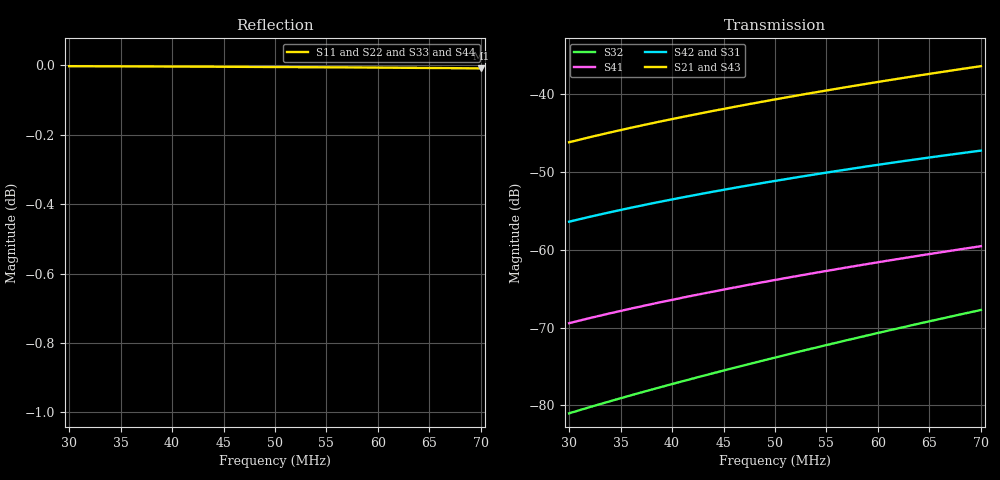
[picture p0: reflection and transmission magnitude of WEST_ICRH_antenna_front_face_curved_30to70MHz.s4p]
! Touchstone file exported from HFSS 2020.2.0
!  File:  C:/Users/JH218595/Documents/ICRH/WEST/HFSS_antenna_front_face/WEST_ICRH_front_face.aedt
!  Generated:  10:17:14  ao%xFBt 03, 2020
!  Design:  Front Face Curved
!  Project:  WEST_ICRH_front_face
!  Setup:  Setup1
!  Solution:  Sweep_operationnal
! Variables:
!  $epsr_dielectric = 1
!  $shift_X = 50mm
!  dphi = -180deg
!Data is not renormalized
# GHZ S MA
! Terminal data exported
! Port[1] = 1
! Port[2] = 2
! Port[3] = 3
! Port[4] = 4
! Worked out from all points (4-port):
!   4001 points, 30 MHz to 70 MHz, reference per port
!   strongest paths, dB at 30 MHz, 40 MHz, 50 MHz, 60 MHz, 70 MHz:
!     S21: -46.2, -43.2, -40.7, -38.4, -36.4
!     S43: -46.2, -43.2, -40.7, -38.4, -36.4
!     S42: -56.4, -53.5, -51.1, -49.1, -47.2
!     S31: -56.4, -53.5, -51.2, -49.1, -47.3
!     S41: -69.4, -66.4, -63.9, -61.6, -59.5
!     S32: -81.0, -77.3, -73.9, -70.7, -67.7
!   lowest |S11| = 0.0 dB at 70 MHz (marker M1)
!   |S11| at or under -10 dB: nowhere
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0.03  0.9997 145.8  0.004914 55.0  0.001514 57.7  0.0003374 -131.5
      0.004914 55.0  0.9997 145.6  8.881e-05 84.9  0.001516 57.7
      0.001514 57.7  8.881e-05 84.9  0.9997 145.6  0.004911 55.0
      0.0003374 -131.5  0.001516 57.7  0.004911 55.0  0.9997 145.8
0.03273  0.9997 142.4  0.005435 51.6  0.001669 54.6  0.0003734 -135.5
         0.005435 51.6  0.9997 142.3  0.0001005 83.8  0.001671 54.6
         0.001669 54.6  0.0001005 83.8  0.9997 142.3  0.005432 51.6
         0.0003734 -135.5  0.001671 54.6  0.005432 51.6  0.9997 142.4
0.04124  0.9996 131.7  0.007196 40.6  0.002183 44.5  0.0004954 -148.5
         0.007196 40.6  0.9996 131.5  0.0001441 79.4  0.002186 44.5
         0.002183 44.5  0.0001441 79.4  0.9996 131.5  0.007192 40.6
         0.0004954 -148.5  0.002186 44.5  0.007192 40.6  0.9996 131.7
0.04964  0.9994 120.3  0.009173 29.0  0.002743 33.8  0.0006331 -162.0
         0.009173 29.0  0.9994 120.1  0.0002 73.5  0.002747 33.8
         0.002743 33.8  0.0002 73.5  0.9994 120.1  0.009168 29.0
         0.0006331 -162.0  0.002747 33.8  0.009168 29.0  0.9994 120.3
0.06046  0.9992 104.4  0.01214 12.8  0.003549 18.9  0.0008407 179.1
         0.01214 12.8  0.9992 104.2  0.0002966 63.4  0.003555 18.9
         0.003549 18.9  0.0002966 63.4  0.9992 104.2  0.01213 12.8
         0.0008407 179.1  0.003555 18.9  0.01213 12.8  0.9992 104.4
0.06535  0.9991 96.7  0.01364 4.9  0.003943 11.7  0.0009466 170.0
         0.01364 4.9  0.9991 96.5  0.0003511 57.8  0.00395 11.7
         0.003943 11.7  0.0003511 57.8  0.9991 96.5  0.01363 4.9
         0.0009466 170.0  0.00395 11.7  0.01363 4.9  0.9991 96.7
0.07  0.999 89.0  0.01515 -2.9  0.004332 4.5  0.001054 161.0
      0.01515 -2.9  0.999 88.8  0.0004101 52.0  0.00434 4.4
      0.004332 4.5  0.0004101 52.0  0.999 88.8  0.01514 -2.9
      0.001054 161.0  0.00434 4.4  0.01514 -2.9  0.999 89.0
